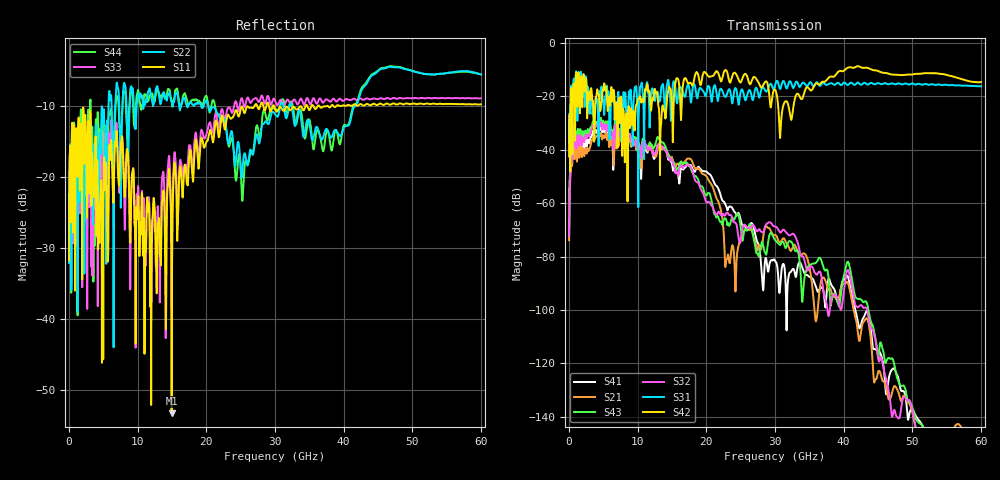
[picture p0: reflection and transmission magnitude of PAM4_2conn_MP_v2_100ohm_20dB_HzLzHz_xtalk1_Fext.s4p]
! Info: Touchstone file created by Circ.  Input file=FAB50GbE_2conn_Midplane_Examax_Topo2_v2_100ohm_20dB_HzLzHz.circ
# Hz S RI R 50
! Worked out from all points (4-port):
!   6000 points, 10 MHz to 60 GHz, reference 50 ohm
!   strongest paths, dB at 10 MHz, 15.01 GHz, 30.01 GHz, 45.01 GHz, 60 GHz:
!     S42: -42.5, -25.2, -17.5, -10.5, -14.7
!     S31: -42.0, -19.1, -15.8, -15.0, -16.3
!     S32: -72.3, -43.9, -68.8, -117.6, -154.7
!     S43: -72.2, -43.5, -73.9, -118.0, -155.1
!     S21: -73.9, -42.9, -72.0, -123.3, -148.5
!     S41: -68.9, -45.5, -81.7, -115.2, -152.8
!   lowest |S11| = -53.2 dB at 14.96 GHz (marker M1), VSWR 1.00, Z = 50.2 + j0.0799 ohm
!   |S11| at or under -10 dB: start of sweep to 27.01 GHz; 29.87 GHz to 34.45 GHz (4.581 GHz wide, 14.2 % of centre); 36.49 GHz to 37.52 GHz (1.034 GHz wide, 2.79 % of centre)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
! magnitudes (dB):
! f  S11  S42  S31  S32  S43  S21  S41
! 10 MHz  -31.8  -42.5  -42.0  -72.3  -72.2  -73.9  -68.9
! 760 MHz  -13.2  -15.9  -14.4  -39.2  -37.2  -42.7  -39.3
! 3.67 GHz  -22.1  -36.5  -26.7  -31.4  -30.2  -36.1  -33.7
! 14.96 GHz  -53.2  -22.1  -21.1  -43.6  -43.4  -42.7  -44.9
! 22.98 GHz  -11.7  -10.6  -19.4  -63.6  -67.0  -81.0  -61.6
! 30.8 GHz  -10.2  -33.6  -17.1  -71.1  -75.6  -74.7  -89.5
! 60 GHz  -9.8  -14.7  -16.3  -154.7  -155.1  -148.5  -152.8
